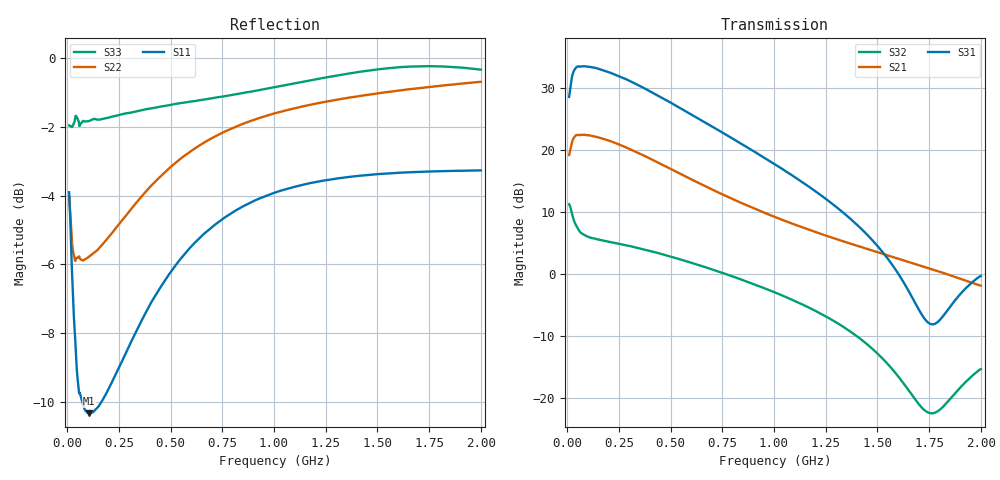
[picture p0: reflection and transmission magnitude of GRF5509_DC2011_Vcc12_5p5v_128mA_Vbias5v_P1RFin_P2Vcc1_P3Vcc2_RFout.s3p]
!Keysight Technologies,N5244B,MY57181157,A.18.40.03
!Date: Wednesday, April 29, 2026 14:22:19
!Correction: S11(C  3-Port  )
!S12(C  3-Port  )
!S13(C  3-Port  )
!S21(C  3-Port  )
!S22(C  3-Port  )
!S23(C  3-Port  )
!S31(C  3-Port  )
!S32(C  3-Port  )
!S33(C  3-Port  )
!S3P File: Measurements: <S11,S12,S13>,
!<S21,S22,S23>,
!<S31,S32,S33>:
# Hz S  dB  R 50
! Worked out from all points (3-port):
!   1991 points, 10 MHz to 2 GHz, reference 50 ohm
!   strongest paths, dB at 10 MHz, 507 MHz, 1.005 GHz, 1.503 GHz, 2 GHz:
!     S31: 28.5, 27.5, 17.7, 4.4, -0.3
!     S21: 19.2, 16.8, 9.2, 3.5, -1.9
!     S32: 11.3, 2.8, -2.9, -12.9, -15.3
!   lowest |S11| = -10.3 dB at 105 MHz (marker M1), VSWR 1.87, Z = 29.7 - j13.9 ohm
!   |S11| at or under -10 dB: 73.05 MHz to 167 MHz (93.92 MHz wide, 78.3 % of centre)
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1e7  -3.90 -55.7  -22.27 -34.2  -57.00 -94.7
     19.17 -137.6  -4.02 -80.3  -31.86 -83.1
     28.54 78.6  11.26 -173.1  -1.96 -110.9
3e7  -7.12 -93.4  -26.75 -43.1  -66.57 150.5
     21.79 -161.9  -5.67 -124.4  -42.85 145.9
     32.49 32.8  8.99 162.4  -1.94 -146.5
4.4e7  -8.77 -111.5  -28.81 -42.8  -65.91 -73.0
       22.37 -172.9  -5.84 -138.3  -42.23 -38.0
       33.29 16.5  7.85 158.7  -1.69 -157.3
1.05e8  -10.34 -135.6  -32.49 -31.9  -72.94 26.1
        22.35 163.6  -5.79 -158.3  -51.09 32.2
        33.38 -16.5  5.97 154.9  -1.83 -169.1
1.73e8  -9.94 -140.7  -33.53 -26.9  -70.76 -134.4
        21.81 146.4  -5.41 -162.6  -45.43 44.0
        32.84 -38.9  5.41 148.5  -1.77 -171.8
2.55e8  -8.96 -141.8  -34.14 -25.8  -65.99 92.8
        20.83 129.1  -4.81 -164.5  -42.40 42.6
        31.81 -60.7  4.87 139.1  -1.65 -172.7
4.78e8  -6.43 -145.9  -35.50 -28.0  -61.52 84.0
        17.32 94.2  -3.29 -169.7  -39.72 31.6
        28.03 -107.6  3.05 113.4  -1.39 -172.9
6.68e8  -5.08 -151.3  -36.55 -29.5  -58.54 83.4
        14.16 74.4  -2.44 -174.7  -39.49 27.2
        24.40 -137.7  1.12 94.1  -1.20 -172.8
1.005e9  -3.91 -160.5  -37.98 -29.6  -54.85 87.2
         9.20 52.1  -1.60 178.2  -40.31 29.7
         17.67 -178.8  -2.94 64.8  -0.84 -173.2
2e9  -3.27 -179.2  -40.87 -41.7  -48.39 91.7
     -1.85 10.0  -0.69 156.3  -35.01 71.3
     -0.28 -126.6  -15.28 123.0  -0.33 172.1
